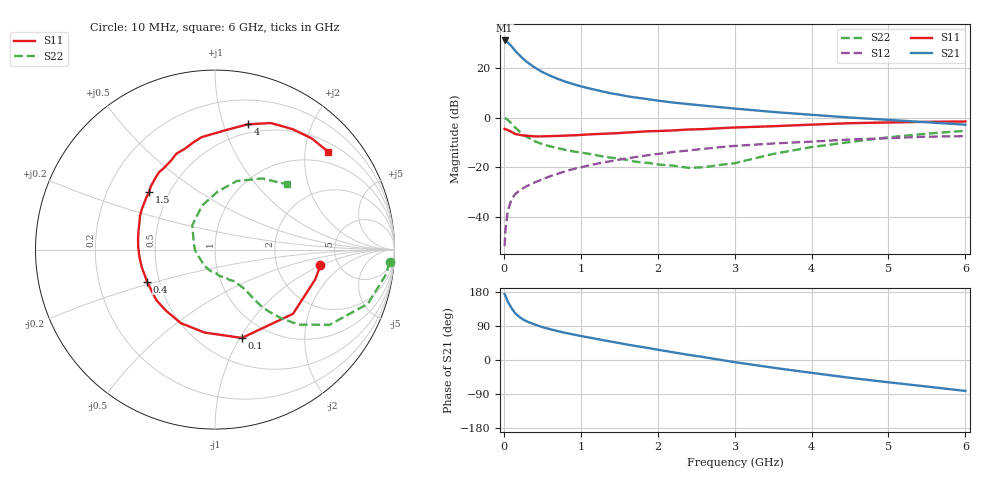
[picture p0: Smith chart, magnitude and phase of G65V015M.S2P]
! SIEMENS Small Signal Semiconductors
! BFG193
! Si NPN RF Bipolar Junction Transistor in SOT223
! VCE = 5 V  IC = 15 mA
! Common Emitter S-Parameters:  August  1996
# GHz  S  MA  R  50
!  f  S11  S21  S12  S22
! GHz  MAG  ANG  MAG  ANG  MAG  ANG  MAG  ANG
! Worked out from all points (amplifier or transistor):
!   36 points, 10 MHz to 6 GHz, reference 50 ohm
!   highest |S21| = 31.0 dB at 10 MHz (marker M1)
!   |S21| within 3 dB of that: start of sweep to 117.7 MHz
!   unconditionally stable (mu >= 1): 780.4 MHz to 2.499 GHz
!   at 250 MHz: K = 0.66, MSG = 26.0 dB, |S12| = -28.4 dB
!   at 1.4 GHz: K = 1.06, MAG = 12.2 dB, |S12| = -17.5 dB
!   at 6 GHz: K = 0.87, MSG = 2.3 dB, |S12| = -7.5 dB
!   S11 on the Smith chart (normalised r, x): 10 MHz: 3.64, -0.99; 100 MHz: 0.76, -1.02; 400 MHz: 0.43, -0.18; 1.5 GHz: 0.39, +0.33; 4 GHz: 0.42, +1.21; 6 GHz: 0.71, +2.52
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0.01  0.5942 -8.5  35.51 174.2  0.0026 88.7  0.9749 -4.2
0.02  0.5825 -16.6  35 169.8  0.0053 89.4  0.9629 -8.2
0.05  0.5631 -39.4  32.64 154.5  0.0129 74.5  0.9039 -19.5
0.1  0.5145 -73.1  27.14 136.8  0.023 64.7  0.7633 -33.3
0.15  0.4657 -97.3  21.86 122.8  0.0292 58.1  0.6272 -41.8
0.2  0.4517 -115.0  18.13 114.1  0.0338 56.6  0.5335 -46.0
0.25  0.4363 -128.9  15.24 106.8  0.0379 55.2  0.4569 -49.0
0.3  0.4315 -139.4  13.1 101.7  0.042 55.7  0.4079 -50.7
0.4  0.4184 -154.8  10.18 93.8  0.0496 56.1  0.3359 -52.1
0.5  0.4197 -166.4  8.241 86.8  0.0574 56.5  0.2922 -52.6
0.6  0.4232 -174.7  6.965 81.4  0.0661 57.0  0.2648 -53.7
0.7  0.4286 177.5  6.019 76.3  0.0743 57.1  0.2429 -55.3
0.9  0.4394 165.6  4.716 67.4  0.092 55.7  0.2096 -57.9
1.1  0.4586 155.5  3.886 59.6  0.1086 53.8  0.1876 -64.4
1.5  0.488 138.8  2.883 44.7  0.1423 47.5  0.1502 -79.7
2.2  0.5514 116.7  2.004 20.4  0.2025 34.4  0.1081 -123.2
2.8  0.6102 101.3  1.623 0.9  0.2533 21.8  0.1113 -178.6
3.5  0.67 84.5  1.298 -20.3  0.3013 5.4  0.1857 133.0
4  0.7215 75.3  1.139 -33.9  0.3288 -4.2  0.2552 106.5
4.5  0.7707 66.2  1.002 -47.0  0.3624 -14.4  0.3227 87.5
5.5  0.821 49.0  0.805 -70.1  0.4138 -38.2  0.4752 56.5
6  0.834 40.7  0.72 -81.6  0.4217 -52.0  0.5433 42.0
